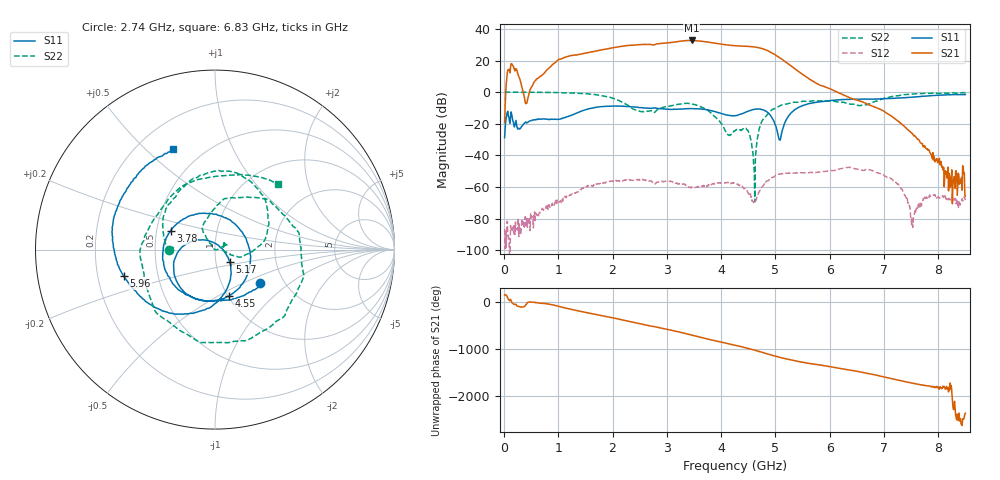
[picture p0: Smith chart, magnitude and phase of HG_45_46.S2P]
!Agilent Technologies,E5071C,MY46523237,B.13.01
!Date: Tue Sep 12 16:47:32 2023
!Data & Calibration Information:
!Freq	S11:SOLT2(ON)	S21:SOLT2(ON)	S12:SOLT2(ON)	S22:SOLT2(ON)
!PortZ  Port1:50+j0  Port2:50+j0
!Above PortZ is port z conversion or system Z0 setting when saving the data.
!When reading, reference impedance value at option line is always used.
# Hz S dB R 50
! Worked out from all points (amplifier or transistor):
!   850 points, 10 MHz to 8.5 GHz, reference 50 ohm
!   highest |S21| = 32.7 dB at 3.46 GHz (marker M1)
!   |S21| within 3 dB of that: 2.37 GHz to 4.15 GHz (1.78 GHz wide, 54.6 % of centre)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
!   unconditionally stable (mu >= 1): 28.33 MHz to 49.27 MHz; 51.31 MHz to end of sweep
!   at 1.42 GHz: K = 5.78, MAG = 32.2 dB, |S12| = -61.6 dB
!   at 4.26 GHz: K = 12.66, MAG = 29.5 dB, |S12| = -57.7 dB
!   at 8.5 GHz: K = 85835.71, MAG = -51.0 dB, |S12| = -68.3 dB
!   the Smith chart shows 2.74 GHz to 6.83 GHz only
!   S11 on the Smith chart (normalised r, x): 2.74 GHz: 1.52, -0.62; 3.78 GHz: 0.59, +0.13; 4.55 GHz: 1.01, -0.56; 5.17 GHz: 1.17, -0.16; 5.96 GHz: 0.31, -0.13; 6.83 GHz: 0.35, +0.61
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1e7  -28.81 -82.5  -19.32 139.6  -86.48 -8.2  0.08 -1.7
1.04e9  -17.00 154.3  20.92 -111.5  -68.52 153.0  -0.32 -170.7
1.43e9  -11.88 137.2  24.20 150.0  -60.87 73.0  -0.83 138.2
1.79e9  -9.14 93.1  26.67 66.2  -57.07 0.7  -2.21 85.0
2.13e9  -8.84 46.6  28.81 -14.9  -56.25 -63.2  -5.58 19.8
2.44e9  -9.47 3.7  29.88 -92.8  -55.19 -113.5  -11.45 -71.0
2.74e9  -10.12 -36.1  29.92 -166.2  -57.33 -171.4  -11.87 -179.8
2.84e9  -10.33 -52.8  30.60 172.7  -56.85 -174.0  -10.93 169.5
3.2e9  -10.74 -102.4  31.95 83.2  -57.90 121.9  -7.71 108.2
3.46e9  -10.43 -143.3  32.67 9.3  -59.76 99.0  -7.50 59.2
3.78e9  -11.40 157.0  31.44 -81.3  -58.93 67.9  -12.20 4.6
4.03e9  -13.79 99.5  30.16 -146.9  -57.27 18.7  -21.20 -16.0
4.26e9  -14.84 25.2  29.32 154.1  -57.71 -33.4  -24.20 37.9
4.55e9  -11.36 -73.3  28.77 71.8  -66.45 -144.8  -30.21 16.0
4.72e9  -10.68 -125.6  27.84 16.2  -61.92 57.7  -20.99 124.8
4.9e9  -14.37 178.3  25.53 -45.4  -54.88 -12.8  -12.22 87.9
5.17e9  -19.51 -39.4  19.54 -128.2  -51.41 -87.5  -7.73 37.3
5.67e9  -6.91 -132.0  7.30 120.1  -50.67 -179.4  -5.58 -41.1
5.96e9  -5.54 -163.6  2.72 69.2  -49.90 136.0  -5.62 -82.0
6.83e9  -4.36 112.6  -9.37 -113.4  -50.16 -60.0  -5.92 46.4
7.09e9  -4.00 87.0  -14.10 177.7  -54.38 -131.1  -3.23 -18.6
8.5e9  -1.46 -105.1  -65.64 152.2  -68.29 -17.2  -0.56 -169.2
